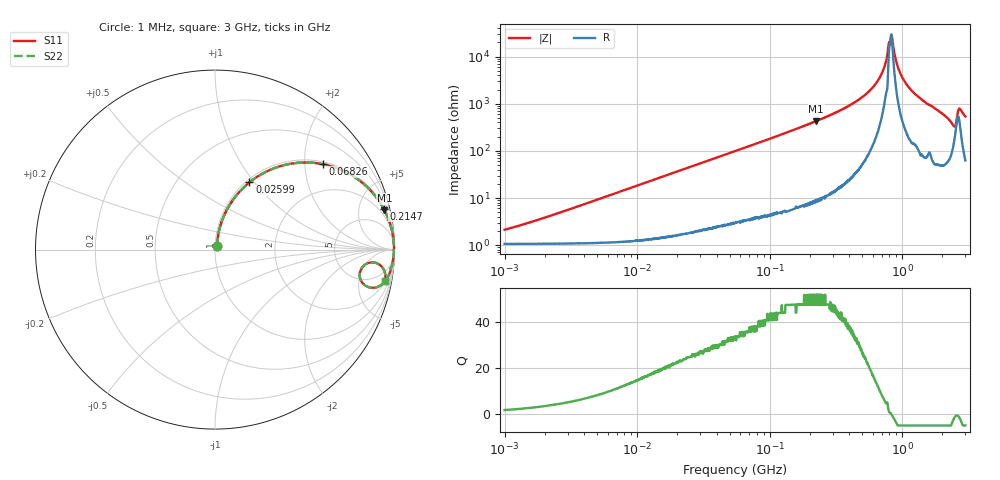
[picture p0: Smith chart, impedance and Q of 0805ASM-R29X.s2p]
!s-Parameter Generated by FASTRON Sdn. Bhd.
!FASTRON P/N : 0805ASM-R29X
!Keysight Technologies: E4991B_MY54100416_A.01.15
!Date: Fri Jun 19 14:51:50 2026
!Version  :Rev00  Fri Jun 19 14:51:50 2026
!Data & Calibration Information:
!Freq  S11  S21  S12  S22
!PortZ  Port1:50+j0  Port2:50+j0
!When reading reference impedance value at option line is always used.
! Remarks : This data is being provided solely for informational purposes.
# Hz S dB R 50
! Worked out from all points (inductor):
!   1601 points, 1 MHz to 3 GHz, reference 50 ohm
!   read as one part in series: L = 293 nH near 1.751 MHz
!   highest Q = 52 at 224.6 MHz (marker M1), where L = 303 nH
!   self-resonance near 825 MHz
!   S11 on the Smith chart (normalised r, x): 1 MHz: 1.02, +0.04; 25.99 MHz: 1.04, +0.94; 68.26 MHz: 1.07, +2.46; 214.7 MHz: 1.17, +8.16; 3 GHz: 2, -11
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1000000  -33.50 58.9  -0.09 -1.0  -0.09 -1.0  -33.50 58.9
3804036  -23.10 77.1  -0.12 -4.0  -0.12 -4.0  -23.10 77.1
1.447069e7  -12.00 72.4  -0.41 -14.6  -0.41 -14.6  -12.00 72.4
2.598685e7  -7.52 62.9  -1.00 -24.9  -1.00 -24.9  -7.52 62.9
5.504702e7  -3.17 44.4  -3.11 -43.9  -3.11 -43.9  -3.17 44.4
6.826239e7  -2.32 38.5  -4.12 -49.9  -4.12 -49.9  -2.32 38.5
2.083556e8  -0.32 14.2  -12.20 -74.6  -12.20 -74.6  -0.32 14.2
2.147061e8  -0.30 13.7  -12.50 -75.1  -12.50 -75.1  -0.30 13.7
2.245966e8  -0.27 13.1  -12.90 -75.8  -12.90 -75.8  -0.27 13.1
4.013235e8  -0.08 6.2  -19.40 -82.3  -19.40 -82.3  -0.08 6.2
5.753936e8  -0.03 2.9  -25.90 -84.1  -25.90 -84.1  -0.03 2.9
7.099691e8  -0.03 1.2  -33.50 -81.4  -33.50 -81.4  -0.03 1.2
7.463997e8  -0.02 0.8  -36.90 -78.1  -36.90 -78.1  -0.02 0.8
7.925923e8  -0.03 0.2  -45.70 -53.5  -45.70 -53.5  -0.03 0.2
8.12673e8  -0.04 0.1  -46.60 -27.3  -46.60 -27.3  -0.04 0.1
8.332625e8  -0.03 -0.1  -49.10 18.3  -49.10 18.3  -0.03 -0.1
9.682285e8  -0.03 -1.3  -32.90 80.5  -32.90 80.5  -0.03 -1.3
1.231095e9  -0.06 -3.4  -24.60 81.8  -24.60 81.8  -0.06 -3.4
2.050964e9  -0.24 -9.5  -15.60 75.7  -15.60 75.7  -0.24 -9.5
2.407135e9  -0.95 -13.7  -12.10 58.7  -12.10 58.7  -0.95 -13.7
2.714296e9  -0.58 -5.9  -18.50 54.0  -18.50 54.0  -0.58 -5.9
3e9  -0.33 -10.3  -14.90 73.0  -14.90 73.0  -0.33 -10.3
